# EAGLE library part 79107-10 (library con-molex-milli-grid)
RECEPTACAL
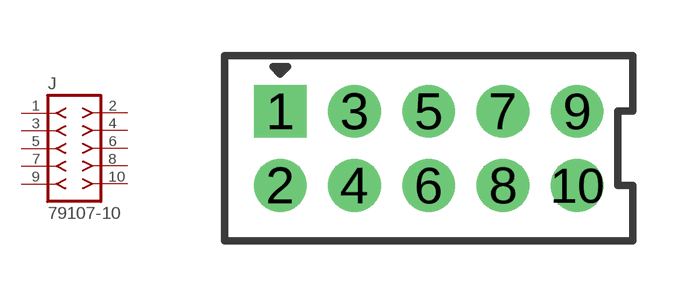
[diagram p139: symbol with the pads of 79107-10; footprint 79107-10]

Designator prefix J

## 79107-10  [79107-10]
1  1  pas
2  2  pas
3  3  pas
4  4  pas
5  5  pas
6  6  pas
7  7  pas
8  8  pas
9  9  pas
10  10  pas

## Footprint 79107-10 (pad centres in mm)
RECEPTACAL Dual Row, Vertical, Through-Hole
drill 0.914 square: 1 -4,1
drill 0.914: 2 -4,-1; 3 -2,1; 4 -2,-1; 5 0,1; 6 0,-1; 7 2,1; 8 2,-1; 9 4,1; 10 4,-1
